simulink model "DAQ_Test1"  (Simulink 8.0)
settings: Solver=FixedStepDiscrete  SolverMode=SingleTasking  StartTime=0  StopTime=inf  FixedStep=dt  RelTol=1e-3  SampleTimeConstraint=Specified
InitFcn:
  | % Sampling Times %
  | dt0=0.001; dt1=0.01; samples=10;
undefined symbols (not defined in the file or in its folder): Volts
libraries: simulink x6, speedgoatlib_IO311 x5, speedgoatlib_IO101 x2

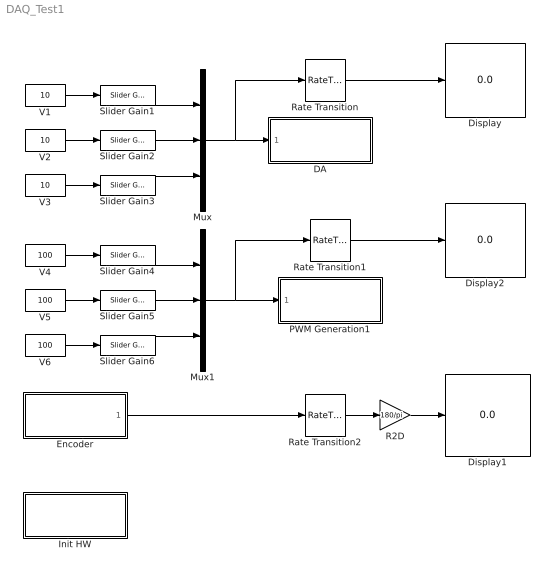
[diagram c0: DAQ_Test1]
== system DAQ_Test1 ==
  DA : Subsystem  TreatAsAtomicUnit=on
  Display : Display
  Display1 : Display
  Display2 : Display
  Encoder : Subsystem  TreatAsAtomicUnit=on
  Init HW : Subsystem  TreatAsAtomicUnit=on
  Mux : Mux  Inputs=3
  Mux1 : Mux  Inputs=3
  PWM Generation1 : Subsystem  TreatAsAtomicUnit=on
  R2D : Gain  Gain=180/pi
  Rate Transition : RateTransition  OutPortSampleTime=dt1
  Rate Transition1 : RateTransition  OutPortSampleTime=dt1
  Rate Transition2 : RateTransition  OutPortSampleTime=dt1
  Slider Gain{1..6} (6 alike) : simulink/Math Operations/Slider Gain  low=-1  gain=0  high=1
  V1 : Constant  Value=10
  V2 : Constant  Value=10
  V3 : Constant  Value=10
  V4 : Constant  Value=100
  V5 : Constant  Value=100
  V6 : Constant  Value=100
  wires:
  Encoder/1(Out1) -> Rate Transition2/1
  V1/1 -> Slider Gain1/1
  Slider Gain1/1 -> Mux/1
  V2/1 -> Slider Gain2/1
  Slider Gain2/1 -> Mux/2
  Rate Transition/1 -> Display/1
  Rate Transition2/1 -> R2D/1
  R2D/1 -> Display1/1
  V3/1 -> Slider Gain3/1
  Slider Gain3/1 -> Mux/3
  Mux/1 -> DA/1(In1), Rate Transition/1
  Rate Transition1/1 -> Display2/1
  V4/1 -> Slider Gain4/1
  V5/1 -> Slider Gain5/1
  V6/1 -> Slider Gain6/1
  Slider Gain4/1 -> Mux1/1
  Slider Gain5/1 -> Mux1/2
  Slider Gain6/1 -> Mux1/3
  Mux1/1 -> PWM Generation1/1(In1), Rate Transition1/1

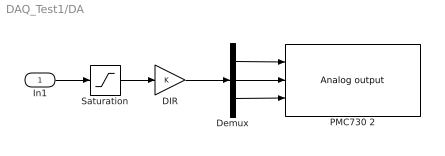
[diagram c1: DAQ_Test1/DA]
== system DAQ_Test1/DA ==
  In1 : Inport
  DIR : Gain
  Demux : Demux  Outputs=3
  PMC730 2 : speedgoatlib_IO101/Analog output  id=1  channel=[1,2,3]  reset=[1,1,1]  initValue=[0,0,0]  ts=dt0  pciSlot=-1
  Saturation : Saturate  UpperLimit=10  LowerLimit=-10
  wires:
  In1/1 -> Saturation/1
  Saturation/1 -> DIR/1
  DIR/1 -> Demux/1
  Demux/1 -> PMC730 2/1
  Demux/2 -> PMC730 2/2
  Demux/3 -> PMC730 2/3

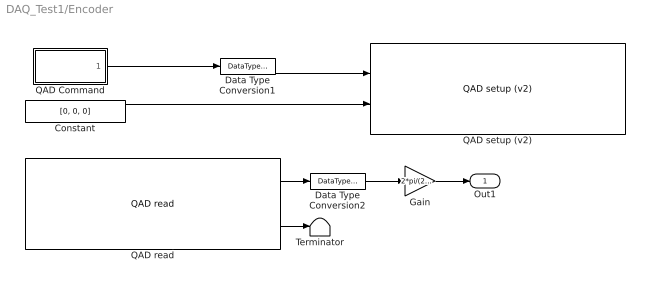
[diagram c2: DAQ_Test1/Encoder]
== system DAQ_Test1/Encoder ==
  Constant : Constant  Value=[0, 0, 0]  OutDataTypeStr=Inherit: Inherit via back propagation
  Data Type Conversion1 : DataTypeConversion  OutDataTypeStr=uint8
  Data Type Conversion2 : DataTypeConversion  OutDataTypeStr=double
  Gain : Gain  Gain=2*pi/(23*2000)
  QAD Command : MATLAB Function  TreatAsAtomicUnit=on
  QAD read : speedgoatlib_IO311/QAD/QAD read  id=1  chan=[1 2 3]  pciSlot=-1  ts=dt0
  QAD setup (v2) : speedgoatlib_IO311/QAD/QAD setup (v2)  id=1  chan=[1,2,3]  debounce=0  quadrature=4x  index=Ignore index input  special=Disabled (cycling counter)  steps=2000  ts=dt0  pciSlot=-1
  Terminator : Terminator
  Out1 : Outport
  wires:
  Gain/1 -> Out1/1
  Constant/1 -> QAD setup (v2)/2
  QAD read/2 -> Terminator/1
  QAD read/1 -> Data Type Conversion2/1
  QAD Command/1(y) -> Data Type Conversion1/1
  Data Type Conversion2/1 -> Gain/1
  Data Type Conversion1/1 -> QAD setup (v2)/1

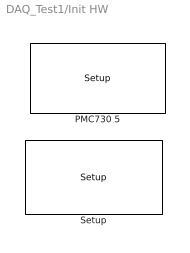
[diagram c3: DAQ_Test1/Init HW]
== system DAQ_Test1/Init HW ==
  PMC730 5 : speedgoatlib_IO101/Setup  group=Analog output setup  id=1  pciSlot=-1  adStartChannel=1  adNumChannel=1  adCoupling=Single-ended  adRange=-10 .. 10 Volts  adAcqMode=Standard  daChannel=[1,2,3]  daReset=[1,1,1]  daInitValue=[0,0,0]  lowerChannel=1  lowerDirection=Input  lowerDIDebounce=0  lowerDOReset=[1]  lowerDOInitValues=[0]  upperChannel=1  upperDirection=Output  upperDIDebounce=0  upperDOReset=0  upperDOInitValues=0
  Setup : speedgoatlib_IO311/Setup/Setup  group=Upper channel group setup  id=1  fpga1=speedgoat_IO311_default  pciSlot=-1  lowerDirection=[1 1 1 1 1 0 0 0 0 0 0 0 1 0 0 0]  lowerReset=[1]  lowerValue=[0]  upperDirection=[1 1 1 1 1 1 1 1 1 0 0 0 0 0 0 0]  upperReset=[1]  upperValue=[0]

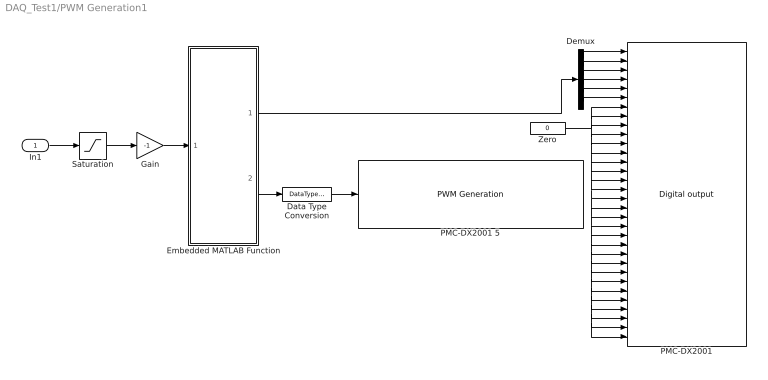
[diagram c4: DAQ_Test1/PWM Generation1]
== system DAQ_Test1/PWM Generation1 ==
  In1 : Inport
  Data Type Conversion : DataTypeConversion  OutDataTypeStr=uint32
  Demux : Demux  Outputs=6
  Embedded MATLAB Function : MATLAB Function  TreatAsAtomicUnit=on
  Gain : Gain  Gain=-1
  PMC-DX2001 : speedgoatlib_IO311/DIO/Digital output  id=1  channelGroup=Upper  portType=32 ports of type double  lowerDirection=[1,1,1,1,1,0,0,0,0,0,0,0,1,0,0,0]  upperDirection=[1,1,1,1,1,1,1,1,1,0,0,0,0,0,0,0]  ts=dt0  pciSlot=-1
  PMC-DX2001 5 : speedgoatlib_IO311/PWM Generation/PWM Generation  channel=[1, 2, 3]  group=Compare count setup  id=1  ts=dt0  pciSlot=-1  initStart=[1]  toggleAStart=[0]  toggleAStop=[0]  toggleBStart=[1]  toggleBStop=[0]  showStart=off  showAStart=off  showAStop=off  showBStart=off  showBStop=off  initA=[5]  initB=[5]  initC=[824]  showA=on  showB=off  showC=off  initActionA=[0,0,1,2]'  initActionB=[0,0,2,1]'  showActionA=off  showActionB=off  triggerSource=[1]  triggerPulseLength=32  protection=[0]
  Saturation : Saturate  UpperLimit=99.9  LowerLimit=-99.9
  Zero : Constant  Value=0
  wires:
  In1/1 -> Saturation/1
  Saturation/1 -> Gain/1
  Embedded MATLAB Function/2(pwm) -> Data Type Conversion/1
  Gain/1 -> Embedded MATLAB Function/1(u)
  Data Type Conversion/1 -> PMC-DX2001 5/1
  Embedded MATLAB Function/1(do) -> Demux/1
  Demux/1 -> PMC-DX2001/1
  Demux/2 -> PMC-DX2001/2
  Demux/3 -> PMC-DX2001/3
  Demux/4 -> PMC-DX2001/4
  Demux/5 -> PMC-DX2001/5
  Demux/6 -> PMC-DX2001/6
  Zero/1 -> PMC-DX2001/9, PMC-DX2001/7, PMC-DX2001/8, PMC-DX2001/10, PMC-DX2001/11, PMC-DX2001/12, PMC-DX2001/13, PMC-DX2001/14, PMC-DX2001/15, PMC-DX2001/16, PMC-DX2001/17, PMC-DX2001/18, PMC-DX2001/19, PMC-DX2001/20, PMC-DX2001/21, PMC-DX2001/22, PMC-DX2001/23, PMC-DX2001/24, PMC-DX2001/25, PMC-DX2001/26, PMC-DX2001/27, PMC-DX2001/28, PMC-DX2001/29, PMC-DX2001/30, PMC-DX2001/31, PMC-DX2001/32

== matlab function PWM Generation1/Embedded
MATLAB Function ==
function [do, pwm] = fcn(u)

MAX_CH=3;
dir=zeros(MAX_CH,1);
pwm=zeros(MAX_CH,1);

for ch=1:MAX_CH
    if u(ch,1)>=0, dir(ch,1)=1; pwm(ch,1)=u(ch,1);
    else dir(ch,1)=0; pwm(ch,1)=-u(ch,1); end
end

do=[dir(1,1),+1,dir(2,1),+1,dir(3,1),+1]';

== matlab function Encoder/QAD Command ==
function y = fcn()

persistent index

if isempty(index), index=0; end

if index==0
    y=[1,1,1];      %  Reset %
else
    y = [0,0,0];
end

index=index+1;
